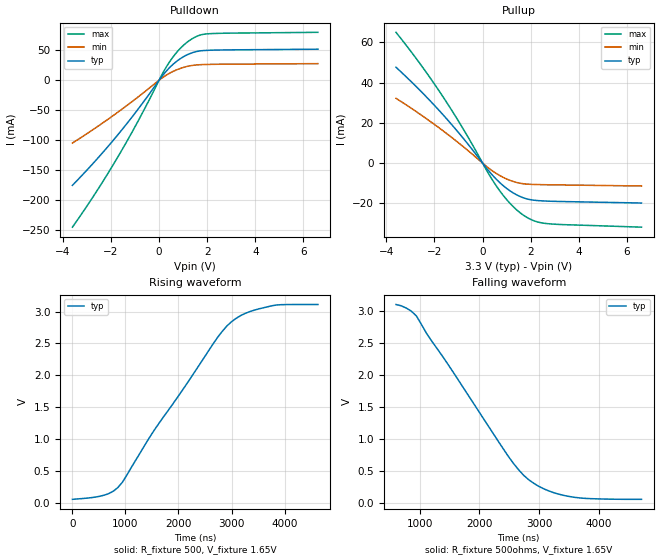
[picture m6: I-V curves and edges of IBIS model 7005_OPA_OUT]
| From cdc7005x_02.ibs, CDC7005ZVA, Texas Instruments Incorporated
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|OPA_OUT
| The operational amplifier is configured as inverting amplifier with
| gain of 1. The input signal is 0V or VCC to achieve HIGH/LOW levels and
| also for voltage/time wave forms.
[Model]   7005_OPA_OUT
Model_type   Output
Polarity   Non-Inverting
Enable   Active-High
Vmeas = 1.65V   |Vref for timing measurements.
Cref = 0pF   |load capacitance for timing spec.
Rref = 500ohms   |500 Ohm to GND.
Vref = 1.65V   |Timing specification test load voltage; GND
|   typ   min   max
C_comp   1.29pF   1.24pF   1.33pF
[Temperature range]   27   125   -20
[Voltage range]   3.3   3.0   3.6
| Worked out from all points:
|   slope of the pulldown table from 0 to 0.495 V, typ, clamps not added: 21.3 ohm
|   slope of the pullup table from 0 to 0.495 V, typ, clamps not added: 69.8 ohm
|   rising waveform, R_fixture 500, V_fixture 1.65V: 20-80 % time 1.47us typ, NA min, NA max; typ from 0.061 V to 3.11 V
|   falling waveform, R_fixture 500ohms, V_fixture 1.65V: 20-80 % time 1.3us typ, NA min, NA max; typ from 3.1 V to 0.058 V
| Notes: (1) Vtable = Vcc - Voutput
|   (2) Pullup data includes the effects of clamping circuitry
[Pullup]
|   27C:3.3V:nominal   125C:3.0V:weak   -20C:3.6V:strong
|  Voltage   I(typ)   I(min)   I(max)
-3.6V     47.68mA    32.25mA    65.05mA
-2.6V     36.16mA    24.32mA    49.43mA
-1.6V     23.46mA    15.68mA    32.15mA
-800mV    12.28mA    8.16mA     16.87mA
200mV     -3.069mA   -1.996mA   -4.281mA
600mV     -8.381mA   -5.36mA    -11.87mA
1V        -12.58mA   -7.883mA   -18.14mA
1.5V      -16.27mA   -9.84mA    -24.11mA
2V        -18.19mA   -10.53mA   -27.97mA
2.3V      -18.61mA   -10.64mA   -29.28mA
2.6V      -18.82mA   -10.72mA   -29.94mA
6.6V      -19.82mA   -11.35mA   -31.81mA
[Pulldown]
|   27C:3.3V:nominal   125C:3.0V:weak   -20C:3.6V:strong
|  Voltage   I(typ)   I(min)   I(max)
-3.6V     -175.2mA   -104.8mA   -244.9mA
-2.6V     -132.3mA   -78.35mA   -185.5mA
-1.6V     -85.4mA    -49.99mA   -120.2mA
-800mV    -44.41mA   -25.68mA   -62.73mA
100mV     5.419mA    3.009mA    7.85mA
300mV     15.15mA    8.398mA    22.04mA
700mV     30.53mA    16.81mA    44.89mA
1.1V      41.04mA    22.34mA    61.21mA
1.3V      44.66mA    24.1mA     67.2mA
1.6V      48.19mA    25.61mA    73.71mA
2V        49.79mA    26.29mA    77.27mA
6.6V      51.69mA    27.64mA    79.82mA
[ramp]
| variable   typ   min   max
dV/dt_r   1.8659/1.4928E-06   NA   NA
dV/dt_f   1.8659/1.3368E-06   NA   NA
[Rising Waveform]
R_fixture = 500
V_fixture =  1.65V
V_fixture_min = 1.5V
V_fixture_max = 1.8V   |  Plot was truncated to
|   allow faster simulation periodes.
|   27C:3.3V:nominal   125C:3.0V:weak  -20C:3.6V:strong
|   Time   V(typ)   V(min)   V(max)
0s        61.3mV     NA         NA
600ns     126.4mV    NA         NA
857.1ns   246.1mV    NA         NA
942.9ns   329.7mV    NA         NA
1.543us   1.144V     NA         NA
2.657us   2.499V     NA         NA
3us       2.84V      NA         NA
3.343us   2.999V     NA         NA
3.771us   3.091V     NA         NA
4.629us   3.11V      NA         NA
[Falling Waveform]
R_fixture = 500ohms
V_fixture =  1.65V
V_fixture_min = 1.5V
V_fixture_max = 1.8V   | Plot was truncated to
|   allow faster simulation periodes.
|   27C:3.3V:nominal   125C:3.0V:weak -20C:3.6V:strong
|   Time   V(typ)   V(min)   V(max)
604.2ns   3.099V     NA         NA
775.6ns   3.044V     NA         NA
947ns     2.92V      NA         NA
1.118us   2.646V     NA         NA
2.49us    724.2mV    NA         NA
2.661us   517mV      NA         NA
2.833us   360.4mV    NA         NA
3.09us    217.8mV    NA         NA
3.518us   100.4mV    NA         NA
4.718us   57.9mV     NA         NA
